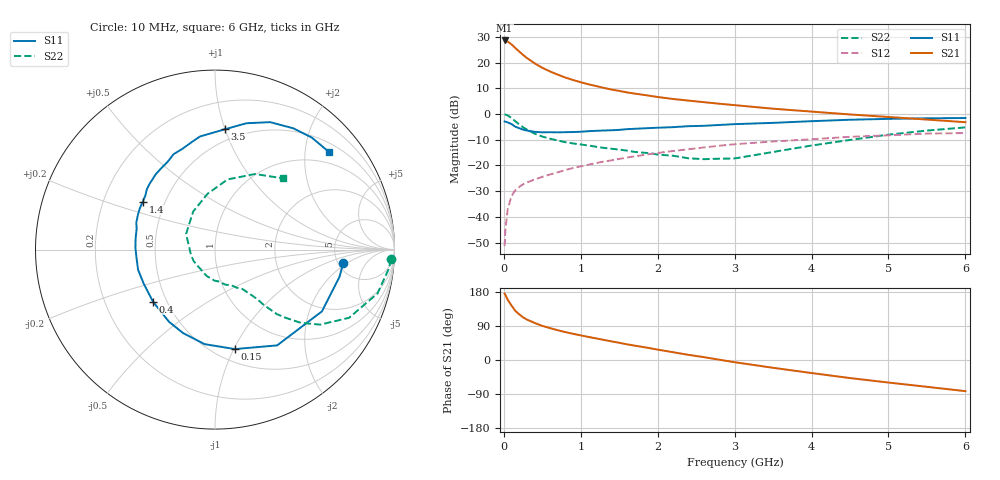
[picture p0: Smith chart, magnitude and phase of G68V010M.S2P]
! SIEMENS Small Signal Semiconductors
! BFG193
! Si NPN RF Bipolar Junction Transistor in SOT223
! VCE = 8 V  IC = 10 mA
! Common Emitter S-Parameters:  August  1996
# GHz  S  MA  R  50
!  f  S11  S21  S12  S22
! GHz  MAG  ANG  MAG  ANG  MAG  ANG  MAG  ANG
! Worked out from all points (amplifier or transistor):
!   36 points, 10 MHz to 6 GHz, reference 50 ohm
!   highest |S21| = 28.6 dB at 10 MHz (marker M1)
!   |S21| within 3 dB of that: start of sweep to 151.4 MHz
!   unconditionally stable (mu >= 1): 922.1 MHz to 2.538 GHz
!   at 250 MHz: K = 0.53, MSG = 25.1 dB, |S12| = -27.3 dB
!   at 1.4 GHz: K = 1.07, MAG = 12.2 dB, |S12| = -18.0 dB
!   at 6 GHz: K = 0.86, MSG = 2.1 dB, |S12| = -7.4 dB
!   S11 on the Smith chart (normalised r, x): 10 MHz: 5.53, -1.74; 150 MHz: 0.62, -1.01; 400 MHz: 0.42, -0.31; 1.4 GHz: 0.38, +0.26; 3.5 GHz: 0.41, +1.00; 6 GHz: 0.70, +2.53
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0.01  0.7182 -6.1  26.88 175.2  0.0027 86.7  0.9819 -3.1
0.02  0.7099 -12.4  26.83 172.0  0.0056 84.7  0.9748 -6.2
0.05  0.688 -30.0  25.6 159.1  0.0139 75.8  0.9379 -15.1
0.1  0.6362 -57.0  22.54 143.6  0.0256 66.4  0.8376 -27.0
0.15  0.5652 -78.7  19.11 129.6  0.0331 58.0  0.7197 -35.5
0.2  0.5299 -96.3  16.39 120.6  0.0382 54.6  0.6303 -40.4
0.25  0.4978 -111.0  14.08 112.6  0.0431 51.8  0.5515 -43.8
0.3  0.4769 -122.5  12.27 106.7  0.0466 51.1  0.4975 -46.2
0.4  0.4512 -140.0  9.67 97.8  0.0534 50.2  0.415 -48.5
0.5  0.4401 -154.6  7.905 90.0  0.0601 50.3  0.3641 -49.6
0.6  0.4431 -165.3  6.722 84.1  0.0668 50.9  0.3315 -50.9
0.7  0.4396 -173.3  5.828 78.6  0.0738 51.6  0.3061 -52.5
0.9  0.4466 172.0  4.576 69.1  0.0892 50.8  0.2678 -55.1
1.1  0.4636 161.0  3.779 60.9  0.1036 50.1  0.2437 -60.5
1.4  0.4829 146.4  2.985 49.2  0.1257 46.9  0.2113 -69.1
1.7  0.5163 135.1  2.492 37.9  0.1503 43.2  0.1834 -79.9
2.2  0.5552 118.5  1.959 20.5  0.1911 34.5  0.1544 -107.4
2.8  0.6119 102.4  1.584 0.8  0.2416 23.1  0.1352 -152.3
3.5  0.6728 85.3  1.268 -20.6  0.2926 7.3  0.1829 151.8
4.5  0.7737 66.6  0.98 -47.7  0.3604 -12.3  0.3134 97.7
5.5  0.825 49.2  0.78 -70.8  0.4169 -36.7  0.4766 62.1
6  0.8359 40.6  0.693 -82.2  0.426 -50.8  0.5495 46.2
